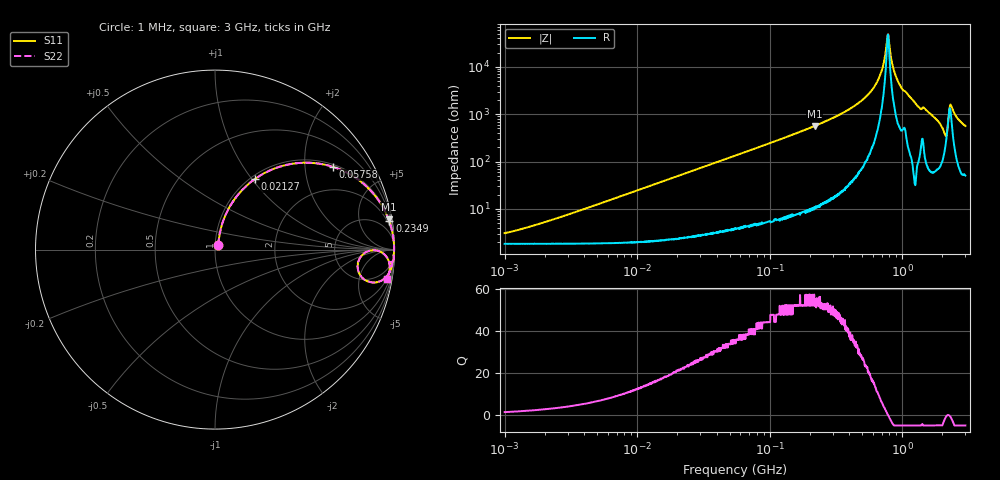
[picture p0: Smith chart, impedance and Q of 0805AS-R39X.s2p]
!s-Parameter Generated by FASTRON Sdn. Bhd.
!FASTRON P/N : 0805AS-R39X
!Keysight Technologies: E4991B_MY54100416_A.01.15
!Date: Mon Jun 15 12:54:46 2026
!Version  :Rev01  Mon Jun 15 12:54:46 2026
!Data & Calibration Information:
!Freq  S11  S21  S12  S22
!PortZ  Port1:50+j0  Port2:50+j0
!When reading reference impedance value at option line is always used.
! Remarks : This data is being provided solely for informational purposes.
# Hz S dB R 50
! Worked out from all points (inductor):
!   1601 points, 1 MHz to 3 GHz, reference 50 ohm
!   read as one part in series: L = 391 nH near 2.249 MHz
!   highest Q = 53.1 at 219 MHz (marker M1), where L = 410 nH
!   self-resonance near 780.8 MHz
!   S11 on the Smith chart (normalised r, x): 1 MHz: 1.04, +0.05; 21.27 MHz: 1.05, +1.04; 57.58 MHz: 1.08, +2.80; 234.9 MHz: 1, +12; 3 GHz: 2, -11
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1000000  -30.40 51.9  -0.16 -1.4  -0.16 -1.4  -30.40 51.9
3804036  -20.60 73.5  -0.20 -5.2  -0.20 -5.2  -20.60 73.5
1.447069e7  -9.67 67.4  -0.68 -19.1  -0.68 -19.1  -9.67 67.4
2.127285e7  -6.87 60.4  -1.20 -26.9  -1.20 -26.9  -6.87 60.4
5.504702e7  -2.04 36.2  -4.58 -52.2  -4.58 -52.2  -2.04 36.2
5.758278e7  -1.90 35.0  -4.83 -53.4  -4.83 -53.4  -1.90 35.0
2.083556e8  -0.18 10.5  -14.80 -78.4  -14.80 -78.4  -0.18 10.5
2.19047e8  -0.16 10.0  -15.20 -79.0  -15.20 -79.0  -0.16 10.0
2.349428e8  -0.14 9.2  -15.90 -79.7  -15.90 -79.7  -0.14 9.2
4.0536e8  -0.04 4.3  -22.40 -84.2  -22.40 -84.2  -0.04 4.3
5.63991e8  -0.02 2.1  -28.90 -85.0  -28.90 -85.0  -0.02 2.1
6.753166e8  -0.02 0.9  -35.90 -82.3  -35.90 -82.3  -0.02 0.9
7.207075e8  -0.02 0.5  -40.80 -76.8  -40.80 -76.8  -0.02 0.5
7.653101e8  -0.02 0.1  -50.40 -47.3  -50.40 -47.3  -0.02 0.1
7.925923e8  -0.02 -0.1  -51.60 38.2  -51.60 38.2  -0.02 -0.1
8.543737e8  -0.02 -0.6  -39.70 77.2  -39.70 77.2  -0.02 -0.6
9.302341e8  -0.02 -1.1  -33.90 81.7  -33.90 81.7  -0.02 -1.1
1.313842e9  -0.06 -3.8  -23.50 82.6  -23.50 82.6  -0.06 -3.8
1.496395e9  -0.08 -4.4  -22.20 80.7  -22.20 80.7  -0.08 -4.4
2.092429e9  -1.10 -11.8  -12.90 52.7  -12.90 52.7  -1.10 -11.8
2.347656e9  -0.32 -3.1  -23.90 54.3  -23.90 54.3  -0.32 -3.1
3e9  -0.27 -9.8  -15.30 75.0  -15.30 75.0  -0.27 -9.8
